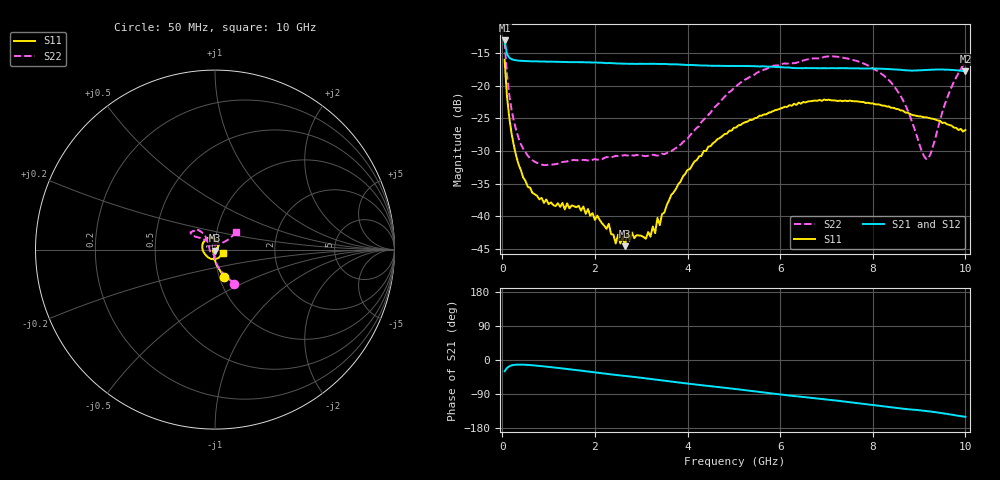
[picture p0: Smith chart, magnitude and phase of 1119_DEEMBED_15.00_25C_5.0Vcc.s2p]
!Hittite Microwave Corp.
!Digital Attenuator/PhaseShifter Rev 1.4.0
!Filename: C:\DATA\DATA\1119_DEEMBED_15.00_25C_5.0Vcc.s2p
!VNA ID: Agilent Technologies,N5224A,MY51441122,A.10.45.03
!Device type:
!2 Port Calibration.
!Temp(C): 25
!Lot Number:
!Serial Number:
!Operator:
!Misc:
!Attenuator:  15.000
# GHZ S DB R 50.0
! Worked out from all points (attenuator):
!   200 points, 50 MHz to 10 GHz, reference 50 ohm
!   highest |S21| = -13.11 dB at 50 MHz (marker M1); lowest = -17.8 dB at 10 GHz (marker M2)
!   lowest |S11| = -44.5 dB at 2.65 GHz (marker M3), VSWR 1.01, Z = 50 - j0.592 ohm
!   |S11| at or under -10 dB: start of sweep to end of sweep
!   |S22| runs from -32.2 to -13.3 dB; largest |S21 - S12| = 0.00039
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0.05  -16.05 -72.2  -13.11 -29.7  -13.11 -29.7  -13.29 -60.9
0.1  -21.56 -84.8  -15.15 -21.4  -15.15 -21.4  -18.21 -75.5
0.2  -27.32 -95.9  -15.97 -14.3  -15.97 -14.3  -23.71 -86.8
0.35  -32.02 -106.1  -16.20 -12.1  -16.20 -12.1  -28.00 -94.0
0.55  -35.49 -118.9  -16.28 -12.9  -16.27 -13.0  -30.71 -100.2
0.9  -37.94 -131.3  -16.33 -16.9  -16.34 -16.9  -32.16 -106.6
1.75  -38.47 -136.2  -16.44 -28.9  -16.45 -28.9  -31.36 -116.0
2.65  -44.55 -91.0  -16.67 -42.1  -16.68 -42.2  -30.62 -141.2
2.7  -42.41 -78.7  -16.67 -42.8  -16.68 -42.9  -30.71 -142.1
3.1  -43.41 -34.6  -16.69 -48.4  -16.71 -48.5  -30.79 -160.9
3.25  -41.54 -11.8  -16.67 -50.7  -16.68 -50.7  -30.57 -168.0
3.3  -42.55 -2.9  -16.69 -51.5  -16.70 -51.6  -30.65 -171.7
3.35  -40.24 2.4  -16.70 -52.2  -16.72 -52.3  -30.73 -174.0
3.4  -41.33 7.5  -16.70 -52.9  -16.71 -53.0  -30.57 -176.3
4  -32.90 41.8  -16.86 -62.1  -16.87 -62.2  -28.09 150.0
5.05  -26.41 72.8  -17.02 -76.8  -17.03 -76.8  -20.11 125.7
6.7  -22.37 123.6  -17.33 -100.1  -17.35 -100.1  -15.86 139.8
7.65  -22.40 157.0  -17.37 -113.6  -17.38 -113.6  -16.22 148.1
8.35  -23.20 -179.3  -17.49 -124.2  -17.49 -124.2  -19.19 142.8
9.2  -24.95 -118.9  -17.60 -135.3  -17.62 -135.3  -31.16 81.8
9.6  -25.91 -76.4  -17.58 -142.3  -17.59 -142.3  -22.01 38.2
10  -26.79 -21.0  -17.82 -150.1  -17.83 -150.1  -16.42 39.6
